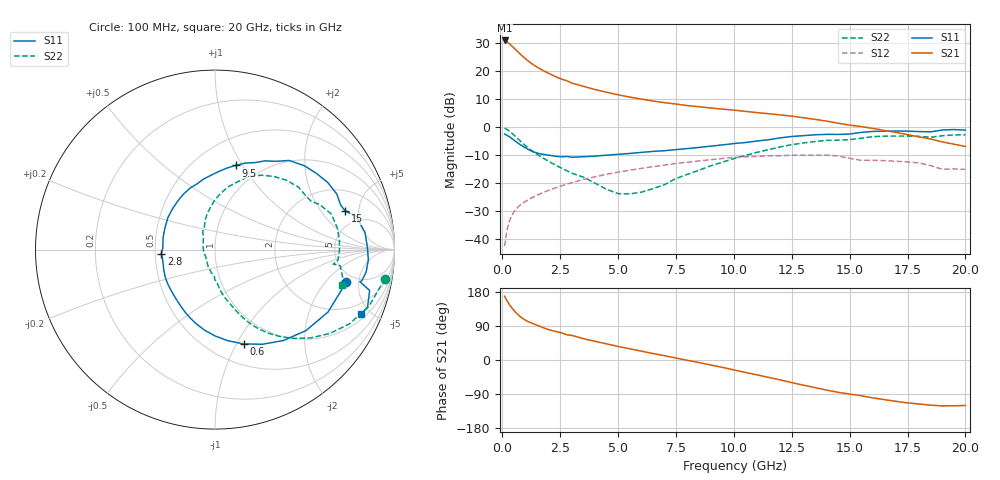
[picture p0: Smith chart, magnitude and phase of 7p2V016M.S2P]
! Infineon Technologies  Discrete & RF Semiconductors
! bfp620
! VCE =  2.0 V,  IC =  16 mA
! Common Emitter S-Parameters:  Sep 2002
# GHz  S  MA  R  50
!  f  S11  S21  S12  S22
! GHz  MAG  ANG  MAG  ANG  MAG  ANG  MAG  ANG
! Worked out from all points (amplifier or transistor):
!   59 points, 100 MHz to 20 GHz, reference 50 ohm
!   highest |S21| = 31.0 dB at 100 MHz (marker M1)
!   |S21| within 3 dB of that: start of sweep to 541.7 MHz
!   unconditionally stable (mu >= 1): 3.599 GHz to 10.09 GHz; 17.14 GHz to end of sweep
!   at 1 GHz: K = 0.63, MSG = 25.5 dB, |S12| = -26.5 dB
!   at 5.5 GHz: K = 1.04, MAG = 11.8 dB, |S12| = -15.4 dB
!   at 20 GHz: K = 1.30, MAG = 0.8 dB, |S12| = -15.1 dB
!   S11 on the Smith chart (normalised r, x): 100 MHz: 4.12, -3.46; 600 MHz: 0.71, -1.07; 2.8 GHz: 0.54, -0.03; 9.5 GHz: 0.76, +0.93; 15 GHz: 3.50, +3.52; 20 GHz: 1.29, -4.39
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0.1  0.7539 -13.9  35.48 168.2  0.0075 69.6  0.9608 -9.7
0.2  0.7195 -28.9  33.38 156.5  0.0146 72.4  0.9137 -20.3
0.3  0.6787 -41.6  31.03 146.8  0.0207 69.5  0.8559 -28.9
0.4  0.6341 -53.0  28.55 138.4  0.026 66.0  0.7918 -36.2
0.5  0.5898 -63.4  26.1 131.0  0.0306 63.0  0.7265 -42.6
0.6  0.549 -73.1  23.8 124.3  0.0347 60.4  0.6639 -48.2
0.7  0.5126 -82.0  21.7 118.4  0.0383 58.4  0.6062 -53.1
0.9  0.4525 -97.4  18.18 108.9  0.0446 55.6  0.5084 -60.8
1  0.4276 -103.9  16.74 105.1  0.0475 54.7  0.468 -63.8
1.2  0.3866 -115.4  14.38 99.1  0.0529 53.5  0.4015 -68.2
1.5  0.3462 -130.1  11.86 91.7  0.0609 52.1  0.3282 -73.3
1.9  0.3214 -147.1  9.644 82.3  0.0718 50.2  0.2599 -79.7
2.8  0.3002 -175.8  6.736 66.4  0.0968 45.2  0.1665 -90.7
3.5  0.2971 166.7  5.383 56.3  0.1164 40.2  0.1281 -99.7
5  0.3276 136.6  3.798 35.8  0.1575 28.0  0.0651 -142.8
7  0.3801 105.1  2.746 11.4  0.2108 10.3  0.0941 133.0
9.5  0.4828 76.3  2.107 -19.4  0.276 -15.3  0.2371 96.1
10.5  0.5334 65.3  1.918 -32.9  0.2961 -27.7  0.3131 84.5
13.5  0.7314 30.7  1.382 -72.8  0.3172 -62.7  0.5549 44.1
15  0.7558 16.6  1.091 -89.8  0.2783 -83.5  0.5993 26.7
17  0.8563 -3.8  0.809 -109.1  0.2467 -94.2  0.6954 4.6
20  0.8886 -23.8  0.453 -120.1  0.1763 -104.8  0.7323 -15.4
